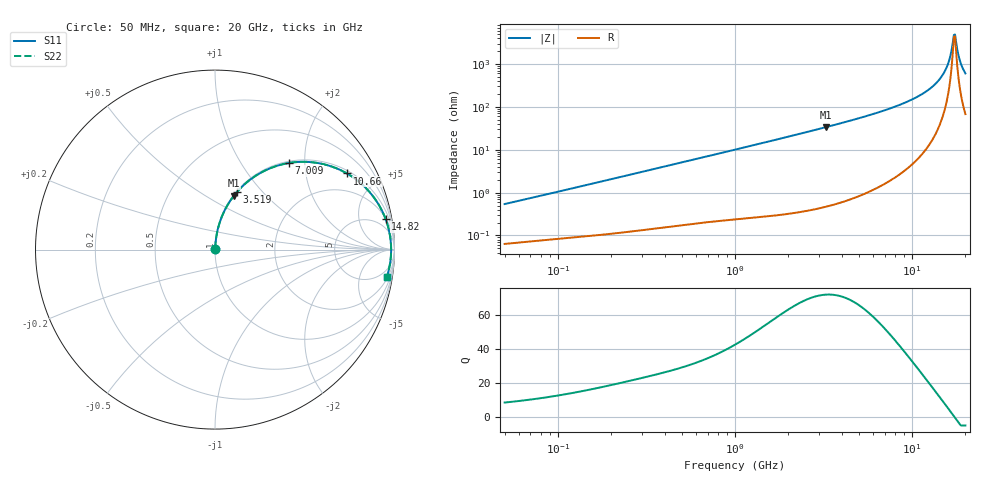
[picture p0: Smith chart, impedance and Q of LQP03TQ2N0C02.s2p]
!Murata Part Number: LQP03TQ2N0C02
!These Parameters are Measured in Series Mode Connection
!  o--[Z]--o
!Port1  Port2
!  o-------o
!Freq. Start=50[MHz] Stop=20[GHz], 401[Steps]
# Hz S RI R 50
!Freq.(Hz) S11(Real) S11(Imag) S21(Real) S21(Imag) S12(Real) S12(Imag) S22(Real) S22(Imag)
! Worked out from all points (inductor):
!   401 points, 50 MHz to 20 GHz, reference 50 ohm
!   read as one part in series: L = 1.69 nH near 51.52 MHz
!   highest Q = 71.8 at 3.265 GHz (marker M1), where L = 1.64 nH
!   self-resonance near 17.22 GHz
!   S11 on the Smith chart (normalised r, x): 50 MHz: 1.00, +0.01; 3.519 GHz: 1.01, +0.73; 7.009 GHz: 1.03, +1.66; 10.66 GHz: 1.12, +3.40; 14.82 GHz: 2, +11; 20 GHz: 2, -12
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5e7  0.000664 0.00536  0.9993 -0.00536  0.9993 -0.00536  0.000664 0.00536
1.364002e8  0.00113 0.0141  0.9989 -0.0141  0.9989 -0.0141  0.00113 0.0141
3.721004e8  0.00291 0.0376  0.9971 -0.0376  0.9971 -0.0376  0.00291 0.0376
1e9  0.0122 0.0988  0.9878 -0.0988  0.9878 -0.0988  0.0122 0.0988
2.728004e9  0.0749 0.2562  0.9251 -0.2562  0.9251 -0.2562  0.0749 0.2562
3.265178e9  0.105 0.2996  0.895 -0.2996  0.895 -0.2996  0.105 0.2996
3.519108e9  0.1208 0.319  0.8792 -0.319  0.8792 -0.319  0.1208 0.319
5.041459e9  0.2337 0.4156  0.7663 -0.4156  0.7663 -0.4156  0.2337 0.4156
7.009217e9  0.4106 0.4824  0.5894 -0.4824  0.5894 -0.4824  0.4106 0.4824
7.442007e9  0.4515 0.4875  0.5485 -0.4875  0.5485 -0.4875  0.4515 0.4875
1.066139e10  0.7357 0.4241  0.2643 -0.4241  0.2643 -0.4241  0.7357 0.4241
1.295331e10  0.8804 0.2974  0.1196 -0.2974  0.1196 -0.2974  0.8804 0.2974
1.482269e10  0.9502 0.1714  0.0498 -0.1714  0.0498 -0.1714  0.9502 0.1714
1.597544e10  0.9726 0.0919  0.0274 -0.0919  0.0274 -0.0919  0.9726 0.0919
1.646126e10  0.9778 0.059  0.0222 -0.059  0.0222 -0.059  0.9778 0.059
1.696185e10  0.9807 0.0257  0.0193 -0.0257  0.0193 -0.0257  0.9807 0.0257
1.721783e10  0.9814 0.00898  0.0186 -0.00898  0.0186 -0.00898  0.9814 0.00898
1.747767e10  0.9814 -0.00776  0.0186 0.00776  0.0186 0.00776  0.9814 -0.00776
1.774144e10  0.9809 -0.0245  0.0191 0.0245  0.0191 0.0245  0.9809 -0.0245
1.88369e10  0.9731 -0.0908  0.0269 0.0908  0.0269 0.0908  0.9731 -0.0908
1.940974e10  0.9659 -0.1233  0.0341 0.1233  0.0341 0.1233  0.9659 -0.1233
2e10  0.9566 -0.155  0.0434 0.155  0.0434 0.155  0.9566 -0.155
